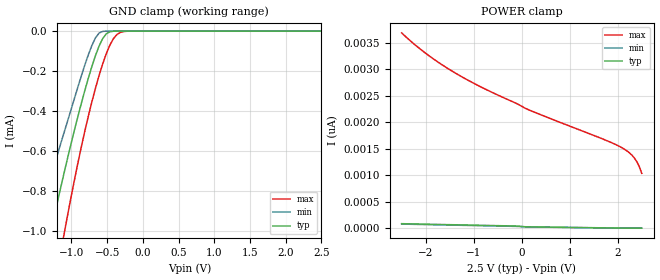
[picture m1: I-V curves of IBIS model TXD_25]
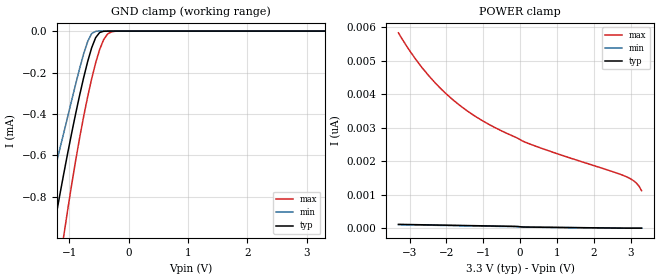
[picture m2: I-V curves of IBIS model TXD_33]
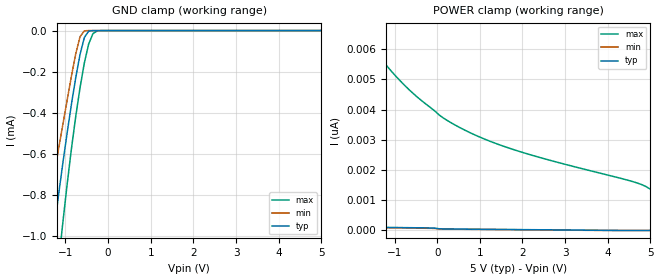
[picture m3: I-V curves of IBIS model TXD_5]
| IBIS file created by Layout Workbench Version 22.1.4.12161.401368   004
| Cadence Design Systems, Inc. 2011
[IBIS ver]   4.2
[File name]  iso6421.ibs
[File Rev]   1.5
[Date]   05 15, 2025
[Source]   Model built from TISPICED simulations at:
   Texas Instruments Incorporated.
   Analog-eLab, HPA 12500 TI Blvd
   Dallas, TX -75243
   For Support e-mail: elab_ibis@list.ti.com
[Notes]   This product is designed as an aid for customers of Texas Instruments.
   No warranties, either expressed or implied, with respect to this third party software (if any)
   or with respect to its fitness for any particular purpose is claimed by Texas Instruments or
   the author. The software (if any) is provided solely on an "as is" basis. The entire risk as to
   its quality and performance is with the customer
[Disclaimer] This product is designed as an aid for customers of Texas Instruments. No warranties, either expressed or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
[Copyright] (C)Copyright 2025 Texas Instruments Incorporated. All rights reserved.
|   ISO6421D
[Component] ISO6421D
[Manufacturer] Texas Instruments Incorporated
[Package]   |8-pin SOIC D package
|   typ   min   max
R_pkg   0.055   0.034   0.067
L_pkg   1.795nH   1.699nH   1.914nH
C_pkg   0.299pF   0.278pF   0.311pF
[Pin]  signal_name   model_name   R_pin   L_pin   C_pin
1   VCC1   POWER   0.067   1.914n   0.278p
2   OUTA   RXD1   0.062   1.816n   0.301p
3   INB   TXD1   0.053   1.699n   0.298p
4   GND1   GND   0.067   1.907n   0.278p
5   GND2   GND   0.034   1.704n   0.311p
6   OUTB   RXD1   0.061   1.808n   0.310p
7   INA   TXD1   0.062   1.817n   0.302p
8   VCC2   POWER   0.034   1.716n   0.311p
|   ISO6421FD
[Component]   ISO6421FD
[Manufacturer]   TI
[Package]   |8 SOIC - D package
|   typ   min   max
R_pkg   0.055   0.034   0.067
L_pkg   1.795nH   1.699nH   1.914nH
C_pkg   0.299pF   0.278pF   0.311pF
[Pin]  signal_name   model_name   R_pin   L_pin   C_pin
1   VCC1   POWER   0.067   1.914n   0.278p
2   OUTA   RXD1   0.062   1.816n   0.301p
3   INB   TXD2   0.053   1.699n   0.298p
4   GND1   GND   0.067   1.907n   0.278p
5   GND2   GND   0.034   1.704n   0.311p
6   OUTB   RXD1   0.061   1.808n   0.310p
7   INA   TXD2   0.062   1.817n   0.302p
8   VCC2   POWER   0.034   1.716n   0.311p
|   ISO6421DWV
[Component]   ISO6421DWV
[Manufacturer]   TI
[Package]   |8 SOIC - DWV package
|   typ   min   max
R_pkg   0.29774   0.1605   0.43022
L_pkg   4.3564E-09   3.8786E-09   4.7833E-09
C_pkg   6.85578E-13   3.7447E-13   1.4026E-12
[Pin]   signal_name   model_name   R_pin   L_pin   C_pin
1   VCC1   POWER   173.13m 4.2001n 0.58836p
2   OUTA   RXD1   426.94m 4.7753n 0.4071p
3   INB   TXD1   430.22m 4.7833n 0.42645p
4   GND1   GND   250.08m 4.5992n 1.4026p
5   GND2   GND   231.29m 4.228n  1.331p
6   OUTB   RXD1   356.74m 4.1895n 0.39605p
7   INA   TXD1   353.02m 4.1972n 0.37447p
8   VCC2   POWER   160.5m  3.8786n 0.55859p
|   ISO6421FDWV
[Component]   ISO6421FDWV
[Manufacturer]   TI
[Package]   |8 SOIC - DWV package
|   typ   min   max
R_pkg   0.29774   0.1605   0.43022
L_pkg   4.3564E-09   3.8786E-09   4.7833E-09
C_pkg   6.85578E-13   3.7447E-13   1.4026E-12
[Pin]   signal_name   model_name   R_pin   L_pin   C_pin
1   VCC1   POWER   173.13m 4.2001n 0.58836p
2   OUTA   RXD1   426.94m 4.7753n 0.4071p
3   INB   TXD2   430.22m 4.7833n 0.42645p
4   GND1   GND   250.08m 4.5992n 1.4026p
5   GND2   GND   231.29m 4.228n  1.331p
6   OUTB   RXD1   356.74m 4.1895n 0.39605p
7   INA   TXD2   353.02m 4.1972n 0.37447p
8   VCC2   POWER   160.5m  3.8786n 0.55859p
|   Model Selectors
[Model Selector] TXD1
TXD_25   TXD Input model for 2.25V - 2.75V
TXD_33   TXD Input model for 3.0V - 3.6V
TXD_5   TXD Input model for 4.5V - 5.5V
[Model Selector] RXD1
RXD_25   RXD Output model for 2.25V - 2.75V
RXD_33   RXD Output model for 3.0V - 3.6V
RXD_5   RXD Output model for 4.5V - 5.5V
[Model Selector] EN
EN_25   TXD Input model for 2.25V - 2.75V
EN_33   TXD Input model for 3.15V - 3.6V
EN_5   TXD Input model for 4.5V - 5.5V
[Model Selector] TXD2
TXDF_25   TXD Input model for 2.25V - 2.75V
TXDF_33   TXD Input model for 3.0V - 3.6V
TXDF_5   TXD Input model for 4.5V - 5.5V
| Models and submodels in the file (12): TXD_25 (Input), TXD_33 (Input), TXD_5 (Input), TXDF_25 (Input), TXDF_33 (Input), TXDF_5 (Input), EN_25 (Input), EN_33 (Input), EN_5 (Input), RXD_25 (3-state), RXD_33 (3-state), RXD_5 (3-state)
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|   TXD_25 Model
[Model]   TXD_25
Model_type   Input
|Signals   TXD
Vinl =  0.750V
Vinh =  1.750V
|   typ   min   max
C_comp   1.3pF   1.1pF   1.5pF
|   typ   min   max
[Temperature Range]   27   -40   125
[Voltage range]   2.5V   2.25V   2.75V
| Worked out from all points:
|   GND clamp passes 1 mA (typ) near -1.29 V on its own axis
[GND_clamp]
|Voltage   I(typ)   I(min)   I(max)
-2.5V     -3.261mA   -2.697mA   -4.025mA
-1.48V    -1.333mA   -1.01mA    -1.787mA
-1.276V   -983uA     -716.4uA   -1.36mA
-1.123V   -739.3uA   -529.9uA   -1.053mA
-1.072V   -661.5uA   -470.4uA   -954.6uA
-919mV    -439.5uA   -290uA     -675.2uA
-766mV    -238.2uA   -120.7uA   -428.7uA
-613mV    -74.62uA   -9.78uA    -221.8uA
-511mV    -13.26uA   -161.8nA   -111.7uA
-409mV    -630.3nA   -1.04nA    -36.14uA
-256mV    -2.009nA   -6.036pA   -1.659uA
2.5V      0A         0A         0A
[POWER_clamp]
|Voltage   I(typ)   I(min)   I(max)
-2.5V     84.61pA    76.91pA    3.684nA
-2.192V   78.79pA    71.19pA    3.438nA
-1.835V   72.09pA    64.59pA    3.191nA
-1.427V   64.46pA    57.09pA    2.951nA
-1.019V   56.88pA    49.63pA    2.744nA
154mV     24.79pA    22.52pA    2.229nA
1.684V    6.302pA    4.156pA    1.684nA
2.092V    1.394pA    0A         1.515nA
2.245V    0A         0A         1.42nA
2.347V    0A         0A         1.323nA
2.449V    0A         0A         1.162nA
2.5V      0A         0A         1.034nA
|   TXD_33 Model
[Model]   TXD_33
Model_type   Input
|Signals   TXD
Vinl =  0.990V
Vinh =  2.310V
|   typ   min   max
C_comp   1.3pF   1.1pF   1.5pF
|   typ   min   max
[Temperature Range]   27   -40   125
[Voltage range]   3.3V   3.0V   3.6V
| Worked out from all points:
|   GND clamp passes 1 mA (typ) near -1.29 V on its own axis
[GND_clamp]
|Voltage   I(typ)   I(min)   I(max)
-3.3V     -4.822mA   -4.059mA   -5.82mA
-1.491V   -1.352mA   -1.027mA   -1.81mA
-1.424V   -1.234mA   -925uA     -1.668mA
-1.29V    -1.006mA   -734.8uA   -1.389mA
-1.223V   -896.7uA   -649.1uA   -1.252mA
-1.089V   -687.3uA   -490.2uA   -987.2uA
-754mV    -223.6uA   -108.8uA   -410.9uA
-620mV    -80.65uA   -12.05uA   -230.3uA
-553mV    -31.67uA   -1.049uA   -153.7uA
-419mV    -886.2nA   -1.734nA   -41.6uA
-218mV    -449.6pA   -6.494pA   -628.3nA
3.3V      0A         0A         0A
[POWER_clamp]
|Voltage   I(typ)   I(min)   I(max)
-3.3V     113.7pA    104.6pA    5.836nA
-3.065V   109.2pA    100.1pA    5.419nA
-2.797V   104pA      95.04pA    4.996nA
-2.328V   94.97pA    86.22pA    4.372nA
-1.792V   84.76pA    76.21pA    3.81nA
-1.256V   74.65pA    66.26pA    3.373nA
-720mV    64.61pA    56.39pA    3.029nA
151mV     33.16pA    30.36pA    2.565nA
2.898V    0A         0A         1.532nA
3.166V    0A         0A         1.339nA
3.233V    0A         0A         1.249nA
3.3V      0A         0A         1.12nA
|   TXD_5 Model
[Model]   TXD_5
Model_type   Input
|Signals   TXD
Vinl =  1.500V
Vinh =  3.500V
|   typ   min   max
C_comp   1.3pF   1.1pF   1.5pF
|   typ   min   max
[Temperature Range]   27   -40   125
[Voltage range]   5.0V   4.5V   5.5V
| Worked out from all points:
|   GND clamp passes 1 mA (typ) near -1.29 V on its own axis
[GND_clamp]
|Voltage   I(typ)   I(min)   I(max)
-5V       -8.158mA   -6.968mA   -9.644mA
-1.465V   -1.306mA   -987uA     -1.755mA
-1.263V   -961.6uA   -699.5uA   -1.333mA
-1.162V   -799.9uA   -575.6uA   -1.13mA
-1.061V   -645uA     -457.5uA   -933.6uA
-758mV    -228.5uA   -112.7uA   -416.8uA
-657mV    -115.6uA   -29.62uA   -276.8uA
-556mV    -33.38uA   -1.189uA   -156.8uA
-455mV    -2.832uA   -10.7nA    -64.96uA
-354mV    -87.76nA   -69.95pA   -14.52uA
-253mV    -1.79nA    -9.666pA   -1.545uA
5V        0A         0A         0A
[POWER_clamp]
|Voltage   I(typ)   I(min)   I(max)
-5V       179.5pA    164pA      20.45nA
-1.868V   115.6pA    102.9pA    6.803nA
-1.767V   113.6pA    101pA      6.576nA
-1.262V   103.8pA    91.4pA     5.583nA
-757mV    94.06pA    81.91pA    4.792nA
51mV      56.19pA    49.29pA    3.815nA
455mV     46.94pA    42.18pA    3.461nA
1.061V    39.62pA    34.91pA    3.053nA
1.768V    31.11pA    26.43pA    2.686nA
2.677V    20.17pA    15.53pA    2.309nA
4.596V    0A         0A         1.612nA
5V        0A         0A         1.364nA
